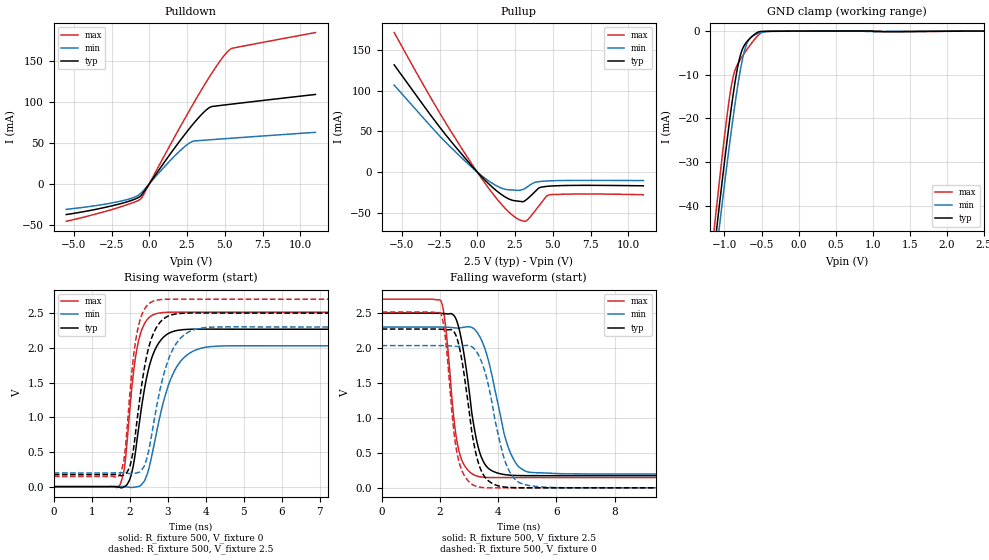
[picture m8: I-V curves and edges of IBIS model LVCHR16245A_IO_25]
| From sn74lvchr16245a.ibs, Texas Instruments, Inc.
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[Model]   LVCHR16245A_IO_25
Model_type  I/O
Vinl=0.7
Vinh=1.7
Enable   Active-Low
Vref =   0
Rref =   500
Cref =   30p
Vmeas =   1.25
| variable   typ   min   max
C_comp   5.33pF   4.75pF   6.48pF
| C_pullup   4.10pF   2.75pF   6.78pF
| C_pulldown   4.60pF   3.27pF   7.14pF
| C_tri-state   5.33pF   4.75pF   6.48pF
[Temperature Range]   40   100   -40
| Ambient temperature   25   85   -40
[Voltage range]   2.5   2.3   2.7
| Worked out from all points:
|   slope of the pulldown table from 0 to 0.375 V, typ, clamps not added: 37.4 ohm
|   slope of the pullup table from 0 to 0.375 V, typ, clamps not added: 50.7 ohm
|   GND clamp passes 1 mA (typ) near -0.61 V on its own axis
|   rising waveform, R_fixture 500, V_fixture 0: 20-80 % time 417ps typ, 573ps min, 291ps max; typ from 0 V to 2.27 V
|   falling waveform, R_fixture 500, V_fixture 2.5: 20-80 % time 505ps typ, 690ps min, 364ps max; typ from 2.5 V to 0.173 V
|   rising waveform, R_fixture 500, V_fixture 2.5: 20-80 % time 392ps typ, 517ps min, 281ps max; typ from 0.173 V to 2.5 V
|   falling waveform, R_fixture 500, V_fixture 0: 20-80 % time 501ps typ, 648ps min, 365ps max; typ from 2.27 V to 0 V
[GND Clamp]
| LVCHR16245A_IO_25
|   Voltage   I(typ)   I(min)   I(max)
-5.5V     -767.3mA   -751.2mA   -793.9mA
-1.15V    -52.02mA   -56.62mA   -47.14mA
-1.125V   -48.25mA   -52.97mA   -43.17mA
-1.1V     -44.51mA   -49.35mA   -39.25mA
-1.075V   -40.81mA   -45.76mA   -35.37mA
-960mV    -24.43mA   -29.74mA   -18.68mA
-885mV    -14.82mA   -20.01mA   -10.67mA
-815mV    -7.658mA   -11.89mA   -7.35mA
-745mV    -3.685mA   -5.548mA   -5.427mA
-630mV    -1.265mA   -1.25mA    -2.666mA
-450mV    -59.9uA    -156.5uA   -99.19uA
2.5V      13.87pA    76.94nA    -1.181nA
[Pulldown]
| LVCHR16245A_IO_25
|   Voltage   I(typ)   I(min)   I(max)
-5.5V     -37.68mA   -31.29mA   -45.91mA
-1.94V    -24.54mA   -21.43mA   -28.49mA
-990mV    -19.03mA   -16.49mA   -22.51mA
-535mV    -14.29mA   -11.04mA   -17.89mA
1.53V     40.06mA    31.18mA    52.39mA
2.695V    68.37mA    50.17mA    90.82mA
2.94V     73.89mA    52.19mA    98.67mA
3.465V    84.81mA    52.97mA    115.1mA
3.995V    93.26mA    53.7mA     131mA
4.8V      95.87mA    54.79mA    153mA
5.345V    97.08mA    55.52mA    164.1mA
11V       109.1mA    62.84mA    184.8mA
[Pullup]
| LVCHR16245A_IO_25
|   Voltage   I(typ)   I(min)   I(max)
-5.5V     131.8mA    106.9mA    171.5mA
-2.525V   56.18mA    45.07mA    73.89mA
-70mV     1.429mA    1.111mA    1.925mA
1.42V     -25.14mA   -18.26mA   -35.67mA
2.065V    -32.82mA   -21.71mA   -48.66mA
2.585V    -35.45mA   -22.39mA   -56.55mA
3.035V    -36.47mA   -21.32mA   -60.19mA
3.255V    -33.9mA    -18.97mA   -59.92mA
4.075V    -19.65mA   -11.82mA   -41.84mA
4.575V    -17.66mA   -10.99mA   -29.92mA
4.82V     -17.27mA   -10.78mA   -27.91mA
11V       -16.89mA   -10.48mA   -27.88mA
[Ramp]
| LVCHR16245A_IO_25
| variable   typ   min   max
dV/dt_r   1.37/4.26E-10   1.22/5.77E-10   1.52/2.96E-10
dV/dt_f   1.40/5.13E-10   1.27/7.38E-10   1.53/3.67E-10
R_load = 500
[Rising Waveform]
| LVCHR16245A_IO_25
R_fixture =   500
C_fixture =   0
L_fixture =   0
V_fixture =   0
V_fixture_min = 0
V_fixture_max = 0
|   Time   V(typ)   V(min)   V(max)
0s        288.2pV    4.207nV    7.489nV
1.74ns    -11.59mV   3.042mV    27.03mV
1.865ns   1.747mV    -319.7uV   303.5mV
2.015ns   132.2mV    -11.37mV   1.208V
2.24ns    878mV      4.03mV     2.126V
2.515ns   1.743V     293mV      2.441V
2.85ns    2.134V     1.15V      2.507V
3.38ns    2.261V     1.835V     2.514V
4.31ns    2.269V     2.025V     2.513V
40ns      2.268V     2.028V     2.513V
[Falling Waveform]
| LVCHR16245A_IO_25
R_fixture =   500
C_fixture =   0
L_fixture =   0
V_fixture =   2.5
V_fixture_min = 2.3
V_fixture_max = 2.7
|   Time   V(typ)   V(min)   V(max)
0s        2.5V       2.3V       2.7V
2.03ns    2.497V     2.3V       2.676V
2.185ns   2.491V     2.299V     2.345V
2.475ns   2.468V     2.29V      1.008V
2.64ns    2.304V     2.286V     553.2mV
3.17ns    877.5mV    2.275V     184.4mV
3.405ns   458.4mV    2.134V     154.6mV
4.36ns    182mV      566.4mV    146.2mV
5.065ns   173.3mV    221.9mV    146.6mV
40ns      173.3mV    197.4mV    146.6mV
[Rising Waveform]
| LVCHR16245A_IO_25
R_fixture =   500
C_fixture =   0
L_fixture =   0
V_fixture =   2.5
V_fixture_min = 2.3
V_fixture_max = 2.7
|   Time   V(typ)   V(min)   V(max)
0s        173.2mV    197.3mV    146.5mV
1.74ns    161.5mV    200mV      175.3mV
1.86ns    175.1mV    196.9mV    447.3mV
2.005ns   302mV      186.4mV    1.367V
2.22ns    1.088V     203.7mV    2.299V
2.475ns   1.958V     470.3mV    2.623V
2.785ns   2.362V     1.374V     2.693V
3.295ns   2.494V     2.116V     2.701V
4.18ns    2.501V     2.299V     2.7V
40ns      2.5V       2.3V       2.7V
[Falling Waveform]
| LVCHR16245A_IO_25
R_fixture =   500
C_fixture =   0
L_fixture =   0
V_fixture =   0
V_fixture_min = 0
V_fixture_max = 0
|   Time   V(typ)   V(min)   V(max)
0s        2.272V     2.034V     2.515V
2.025ns   2.269V     2.035V     2.495V
2.175ns   2.265V     2.034V     2.186V
2.46ns    2.242V     2.027V     878.8mV
2.63ns    2.076V     2.024V     413.7mV
3.135ns   701.9mV    2.008V     41.72mV
3.405ns   258.2mV    1.829V     6.151mV
4.315ns   6.816mV    299mV      -435.2uV
5.255ns   -431.9uV   20.97mV    116.5uV
40ns      49.97uV    112.8uV    16.94uV
